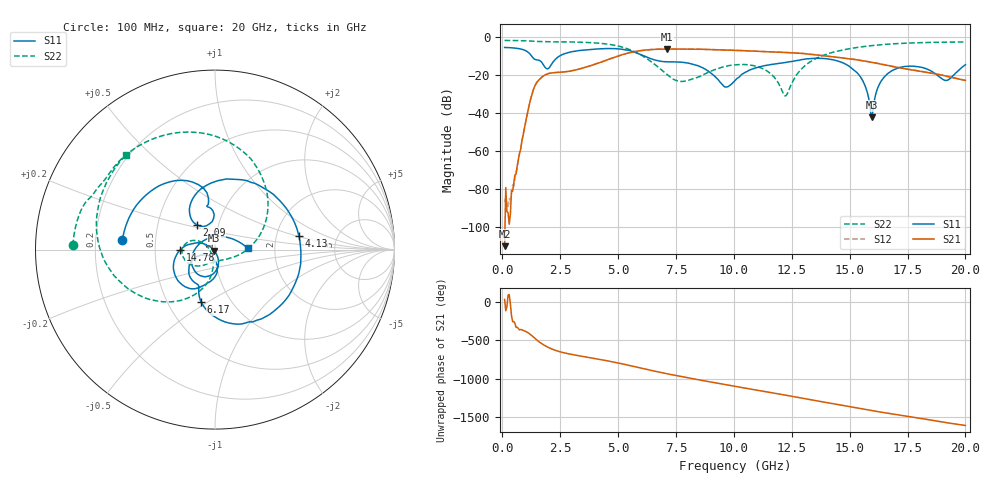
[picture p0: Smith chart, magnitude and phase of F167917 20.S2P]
!  2-Port S-parameters saved by WinCal
! VAR MeasName=S-Parameters (CALIBRATED_DATA) read from VNA (N5242A)
! VAR MeasDate=2016-11-22 9:00:42
! VAR NAME=F167917 20
! VAR FILENAME=F167917 20.S2P
! VAR DATE=2016-11-22 9:00:42
! VAR PHYS_PORTS=1,2
# Hz S DB R 50
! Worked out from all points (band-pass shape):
!   401 points, 100 MHz to 20 GHz, reference 50 ohm
!   highest |S21| = -6.54 dB at 7.115 GHz (marker M1); lowest = -110.3 dB at 100 MHz (marker M2)
!   |S21| within 3 dB of the highest: 5.17 GHz to 13.49 GHz (8.324 GHz wide, 89.2 % of centre)
!   lowest |S11| = -42.4 dB at 15.97 GHz (marker M3), VSWR 1.02, Z = 49.6 - j0.642 ohm
!   |S11| at or under -10 dB: 1.251 GHz to 2.504 GHz (1.253 GHz wide, 66.7 % of centre); 6.086 GHz to end of sweep
!   |S22| runs from -31.2 to -2.0 dB; largest |S21 - S12| = 0.0044
!   S11 on the Smith chart (normalised r, x): 100 MHz: 0.32, +0.05; 2.09 GHz: 0.79, +0.22; 4.13 GHz: 2.69, +0.51; 6.17 GHz: 0.73, -0.47; 14.78 GHz: 0.67, -0.00; 20 GHz: 1.44, +0.02
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1e8  -5.71 174.2  -110.31 34.3  -87.20 33.7  -2.03 178.3
4.98e8  -5.98 150.5  -77.00 105.3  -78.74 120.1  -2.07 171.6
1.3935e9  -11.89 98.5  -26.35 -110.8  -26.33 -110.9  -2.51 156.5
2.09e9  -15.26 126.5  -19.21 112.8  -19.18 112.6  -2.77 147.0
3.43325e9  -7.21 52.4  -16.70 11.4  -16.70 11.2  -2.97 121.5
4.12975e9  -6.49 9.0  -13.99 -25.4  -14.00 -25.4  -3.44 103.5
5.1745e9  -6.65 -56.2  -9.52 -87.0  -9.51 -86.9  -5.49 66.1
6.1695e9  -10.41 -104.8  -7.10 -155.6  -7.07 -155.6  -11.00 21.6
6.7665e9  -12.83 -113.5  -6.62 164.9  -6.60 164.9  -16.42 -7.7
7.11475e9  -13.25 -115.8  -6.54 143.1  -6.53 143.1  -19.93 -27.5
8.3585e9  -14.97 -144.3  -6.60 70.8  -6.56 70.8  -21.83 -113.6
9.60225e9  -26.45 -132.1  -7.02 2.6  -7.03 2.7  -15.76 -150.5
1.005e10  -23.24 -87.1  -7.23 -21.3  -7.23 -21.2  -14.92 -164.5
1.13435e10  -15.24 -96.3  -7.92 -89.6  -7.88 -89.3  -17.46 157.8
1.2239e10  -13.60 -107.4  -8.35 -137.0  -8.32 -137.0  -31.20 -150.1
1.338325e10  -11.49 -130.4  -9.37 160.1  -9.33 160.2  -12.61 -108.7
1.477625e10  -14.18 -179.2  -11.37 85.5  -11.36 85.5  -6.85 -142.2
1.55225e10  -22.28 153.6  -12.65 45.8  -12.66 45.9  -5.38 -157.2
1.597025e10  -42.39 -121.5  -13.57 21.7  -13.58 22.2  -4.72 -165.6
1.67165e10  -18.85 -86.3  -15.33 -16.3  -15.32 -15.6  -3.93 -179.0
1.915425e10  -23.09 103.9  -20.71 -134.3  -20.66 -134.0  -2.92 144.3
2e10  -14.80 2.4  -23.07 -172.4  -22.95 -171.9  -2.82 133.5
